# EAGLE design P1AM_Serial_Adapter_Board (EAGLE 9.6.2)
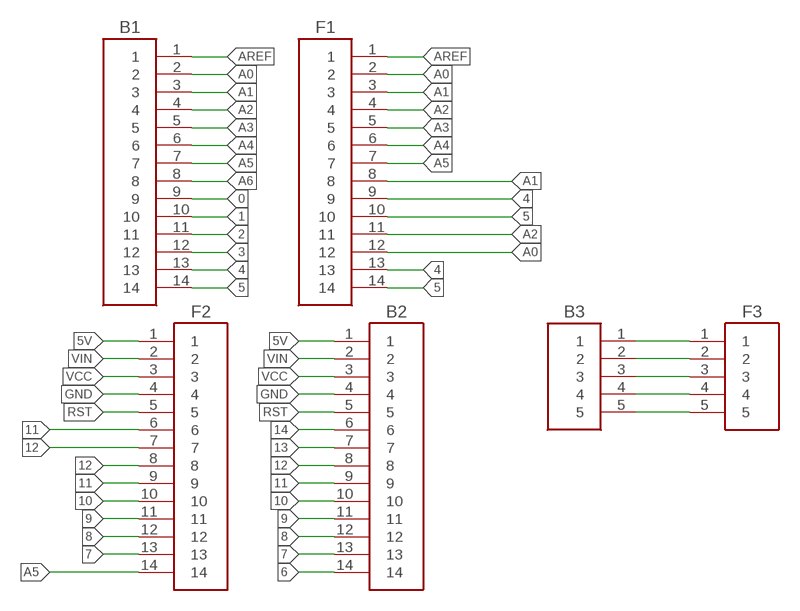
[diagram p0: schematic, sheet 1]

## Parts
B1  14-PN_HDR-2.54  [14-PN_HDR_SMD]
B2  14-PN_HDR-2.54  [14-PN_HDR_SMD]
B3  5-PN_HDR-2.54  [5-PN_HDR_SMD]
F1  14-PN_HDR-2.54  [14-PN_HDR_SMD]
F2  14-PN_HDR-2.54  [14-PN_HDR_SMD]
F3  5-PN_HDR-2.54  [5-PN_HDR_SMD]

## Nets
0: B1.9
1: B1.10
2: B1.11
3: B1.12
4: B1.13 F1.9 F1.13
5: B1.14 F1.10 F1.14
5V: B2.1 F2.1
6: B2.14
7: B2.13 F2.13
8: B2.12 F2.12
9: B2.11 F2.11
10: B2.10 F2.10
11: B2.9 F2.6 F2.9
12: B2.8 F2.7 F2.8
13: B2.7
14: B2.6
A0: B1.2 F1.2 F1.12
A1: B1.3 F1.3 F1.8
A2: B1.4 F1.4 F1.11
A3: B1.5 F1.5
A4: B1.6 F1.6
A5: B1.7 F1.7 F2.14
A6: B1.8
AREF: B1.1 F1.1
GND: B2.4 F2.4
N$1: B3.1 F3.1
N$2: B3.2 F3.2
N$3: B3.3 F3.3
N$4: B3.4 F3.4
N$5: B3.5 F3.5
RST: B2.5 F2.5
VCC: B2.3 F2.3
VIN: B2.2 F2.2

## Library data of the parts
B1 B2 F1 F2 = P1AM:14-PN_HDR-2.54: 2.54mm (0.1") Pitch SIL SMT Pin Header, selective gold + tin, 10 contacts Source: Datasheet
B3 F3 = P1AM:5-PN_HDR-2.54: 2.54mm (0.1") Pitch SIL SMT Pin Header, selective gold + tin, 10 contacts Source: Datasheet

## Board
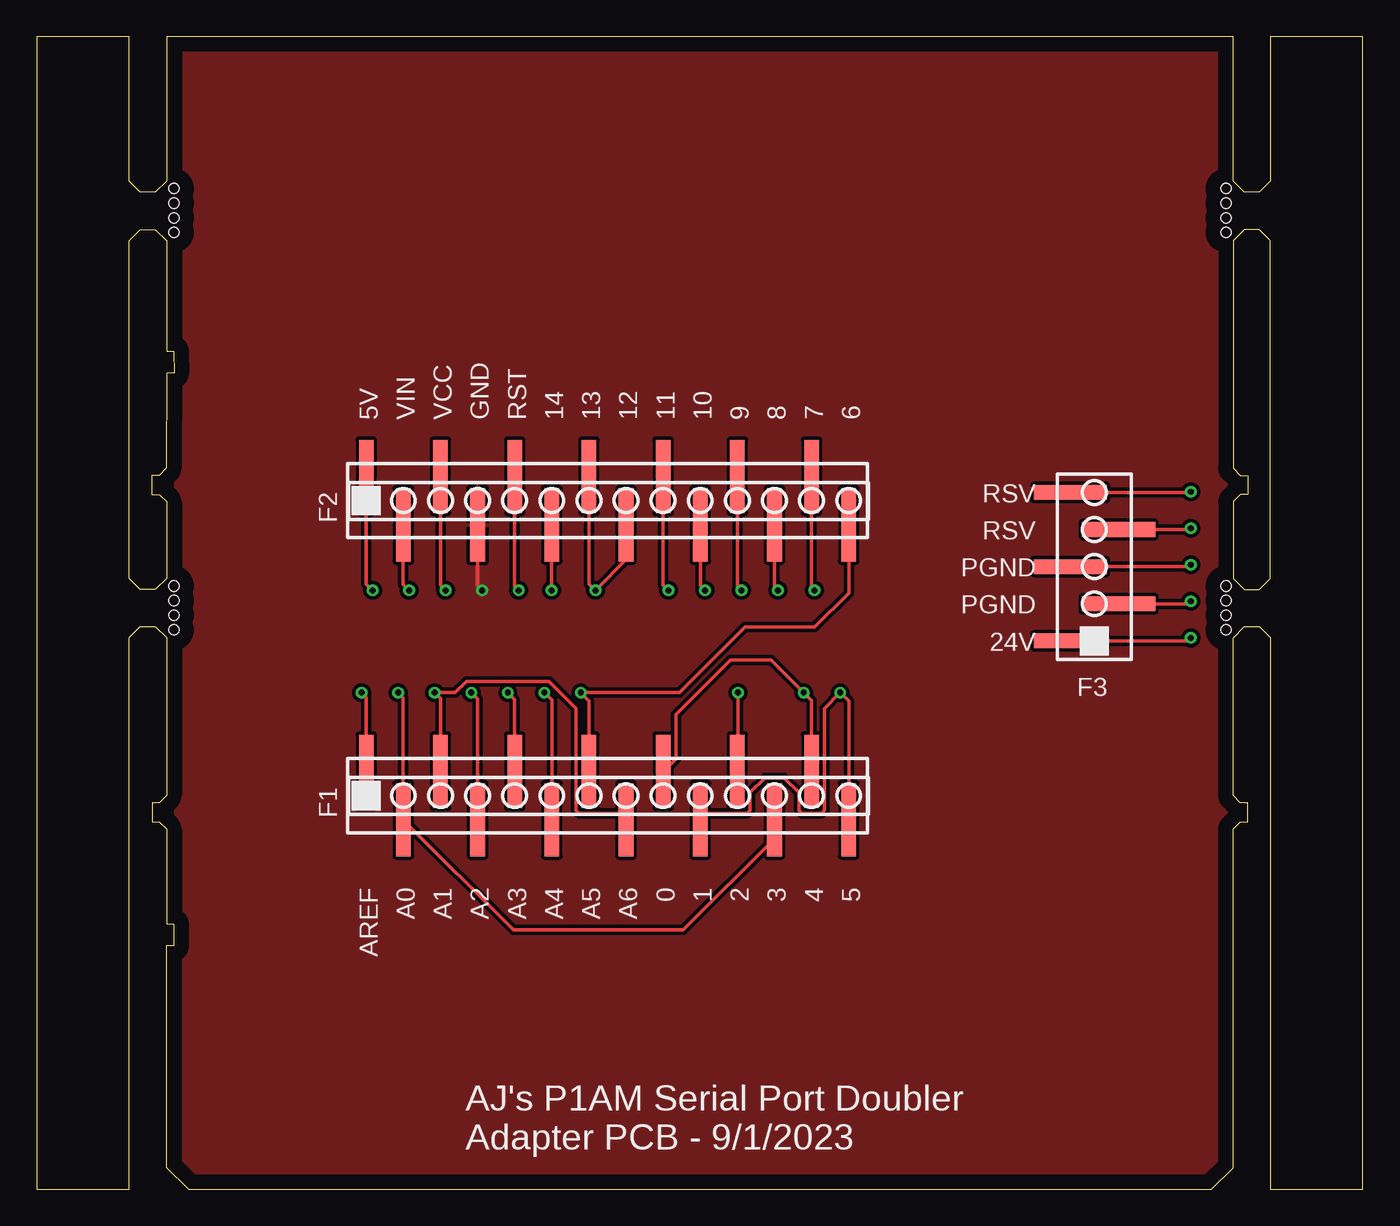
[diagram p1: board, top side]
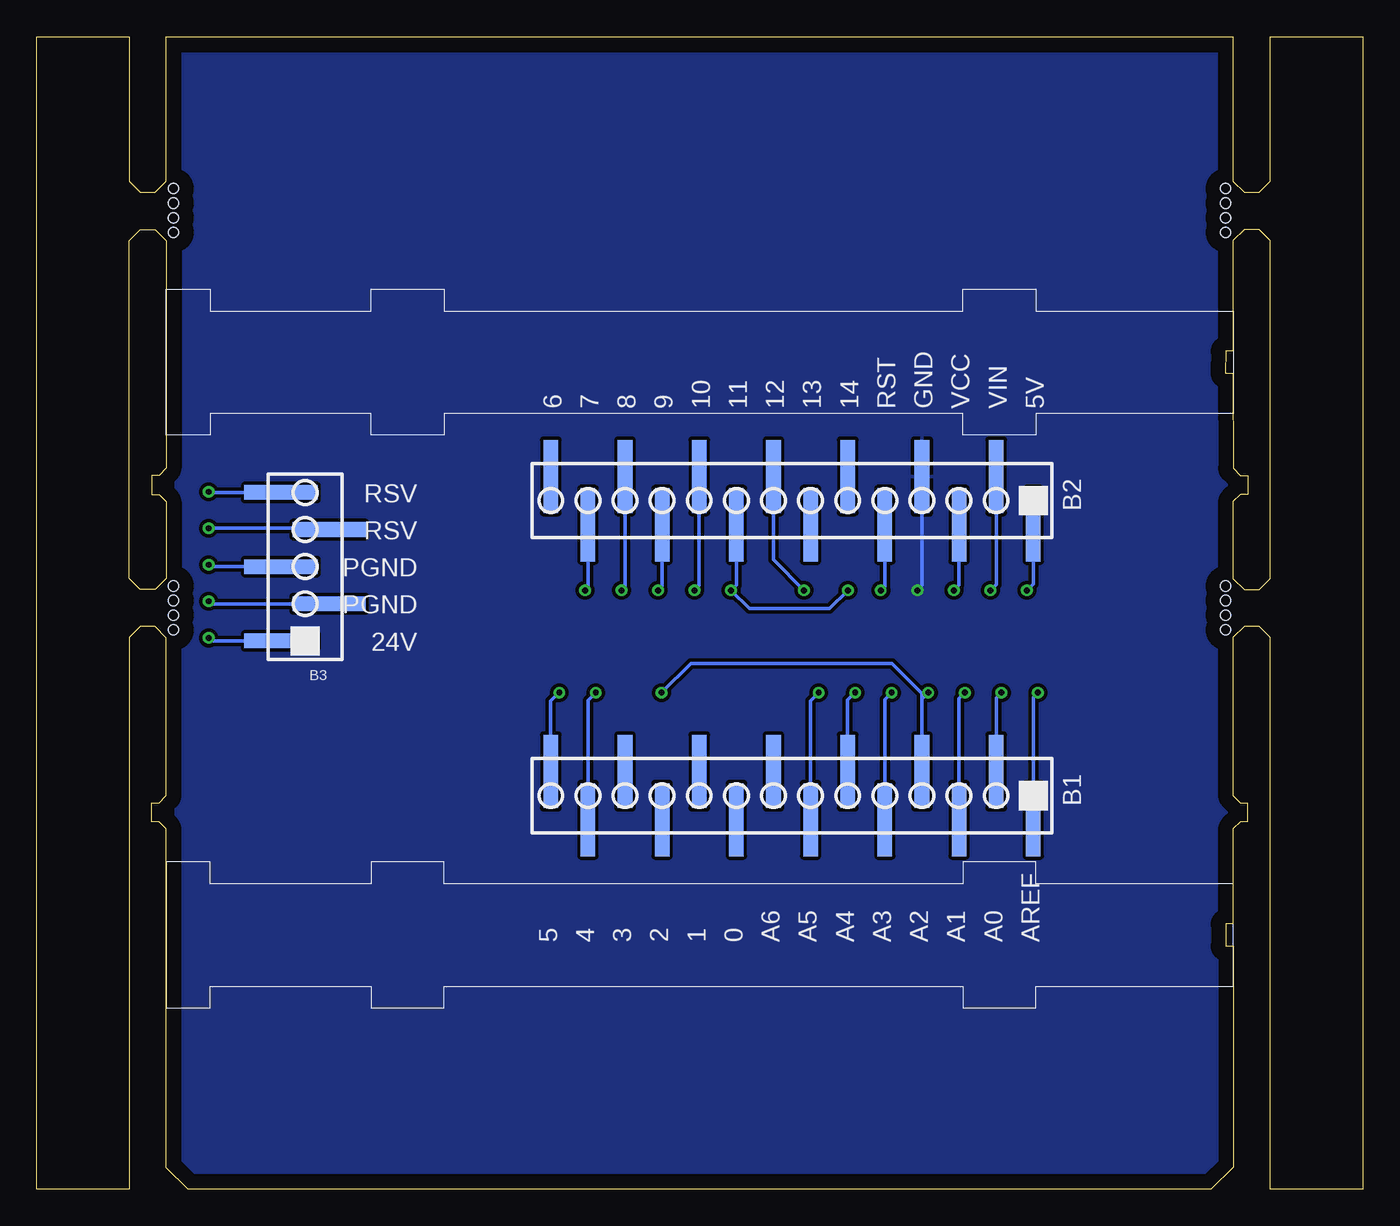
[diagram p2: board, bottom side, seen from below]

Size 90.78 x 78.91 mm. Coordinates in mm from the lower left corner, seen from the top.
Outline: 78 segments
Copper layers (1*16): Top 0.035mm / dielectric 1.5mm / Bottom 0.035mm
Design rules "default *": minimum track width 6mil, minimum drill 0.35mm, track to track 0.24mm, track to pad 0.25mm, pad to pad 0.25mm, via to via 0.25mm, smd to smd 0.2mm, copper to edge 40mil, drill to drill 6mil, minimum pad ring 10mil, minimum via ring 8mil, stop-mask expansion 4mil, vias tented up to drill 0mil, thermal gap 10mil
Holes 0.7 mm at 9.4,68.5 9.4,67.5 9.4,66.5 9.4,65.5 9.4,41.3 9.4,40.3 9.4,39.3 9.4,38.3 81.4,38.3 81.4,39.3 81.4,40.3 81.4,41.3 81.4,65.5 81.4,66.5 81.4,67.5 81.4,68.5

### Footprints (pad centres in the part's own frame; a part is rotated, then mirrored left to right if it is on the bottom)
14-PN_HDR_SMD = smd 1 x 5: 1 0,1.655; 2 2.54,-1.655; 3 5.08,1.655; 4 7.62,-1.655; 5 10.16,1.655; 6 12.7,-1.655; 7 15.24,1.655; 8 17.78,-1.655; 9 20.32,1.655; 10 22.86,-1.655; 11 25.4,1.655; 12 27.94,-1.655; 13 30.48,1.655; 14 33.02,-1.655
5-PN_HDR_SMD = smd 1 x 5: 1 0,1.655; 2 2.54,-1.655; 3 5.08,1.655; 4 7.62,-1.655; 5 10.16,1.655

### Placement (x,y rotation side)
B1  22.57,26.95 180 bottom
B2  22.57,47.14 180 bottom
B3  72.4,37.54 90 bottom
F1  22.57,26.95 0 top
F2  22.57,47.14 0 top
F3  72.4,37.54 90 top

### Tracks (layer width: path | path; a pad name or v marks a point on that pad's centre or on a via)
4  (via drill 0.4)
  Top 0.254: F1.13 53.05,33.45 v52.5,34 50.25,36.25 47.5,36.25 43.75,32.5 43.75,29.47 F1.9
  Bottom 0.254: v52.5,34 53.05,33.45 B1.13
5  (via drill 0.4)
  Top 0.254: F1.14 55.59,33.41 v55,34 53.92,32.92 53.92,25.95 53.7,25.73 52.39,25.73 52.17,25.95 52.17,27.16 51.16,28.17 49.85,28.17 48.84,27.16 48.84,25.95 48.62,25.73 45.86,25.73 F1.10
  Bottom 0.254: v55,34 55.59,33.41 B1.14
5V  (via drill 0.4)
  Top 0.254: v23,41 22.57,41.44 F2.1
  Bottom 0.254: B2.1 22.57,41.44 v23,41
7  (via drill 0.4)
  Top 0.254: F2.13 53.05,41.2 v53.25,41
  Bottom 0.254: v53.25,41 53.05,41.2 B2.13
8  (via drill 0.4)
  Top 0.254: v50.75,41 50.51,41.24 F2.12
  Bottom 0.254: B2.12 50.51,41.24 v50.75,41
9  (via drill 0.4)
  Top 0.254: F2.11 47.97,41.28 v48.25,41
  Bottom 0.254: v48.25,41 47.97,41.28 B2.11
10  (via drill 0.4)
  Top 0.254: v45.75,41 45.42,41.33 F2.10
  Bottom 0.254: B2.10 45.42,41.33 v45.75,41
11  (via drill 0.4)
  Top 0.254: F2.9 42.88,41.37 v43.25,41 | v35.25,41 35.25,45.47 F2.6
  Bottom 0.254: B2.9 42.88,41.37 v43.25,41 42,39.75 36.5,39.75 v35.25,41
12  (via drill 0.4)
  Top 0.254: F2.7 37.8,41.45 v38.25,41 40.34,43.09 F2.8
  Bottom 0.254: v38.25,41 40.34,43.09 B2.8
A0  (via drill 0.4)
  Top 0.254: v24.75,34 25.11,33.65 F1.2 32.65,17.75 44.25,17.75 50.51,24 F1.12
  Bottom 0.254: v24.75,34 25.11,33.65 B1.2
A1  (via drill 0.4)
  Top 0.254: F1.3 27.64,33.6 v27.25,34 28.65,34 29.43,34.78 35.07,34.78 36.93,32.92 36.93,25.95 37.15,25.73 39.91,25.73 F1.8
  Bottom 0.254: B1.3 27.64,33.6 v27.25,34
A2  (via drill 0.4)
  Top 0.254: F1.4 30.18,33.56 v29.75,34 | v48,34 48,28.64 F1.11
  Bottom 0.254: v29.75,34 30.18,33.56 B1.4 30.18,33.94 32.25,36 46,36 v48,34
A3  (via drill 0.4)
  Top 0.254: v32.25,34 32.73,33.52 F1.5
  Bottom 0.254: B1.5 32.73,33.52 v32.25,34
A4  (via drill 0.4)
  Top 0.254: F1.6 35.27,33.48 v34.75,34
  Bottom 0.254: v34.75,34 35.27,33.48 B1.6
A5  (via drill 0.4)
  Top 0.254: F1.7 37.8,33.45 v37.25,34 44,34 48.5,38.5 53.25,38.5 55.59,40.84 F2.14
  Bottom 0.254: B1.7 37.8,33.45 v37.25,34
AREF  (via drill 0.4)
  Top 0.254: v22.25,34 22.57,33.69 F1.1
  Bottom 0.254: B1.1 22.57,33.69 v22.25,34
GND  (via drill 0.4)
  Top 0.254: F2.4 30.18,41.31 v30.5,41
  Bottom 0.254: v30.5,41 30.18,41.31 B2.4
  pour Top: 9.5,78.5 80.75,78.5 81.5,77.75 81.5,69.5 80.5,68.5 80.5,65.5 81.5,64.5 81.5,42.25 80.75,41.5 80.75,38 81.5,37.25 81.5,2 80,0.5 10.75,0.5 9.5,1.75 9.5,37.5 10.25,38.25 10.25,41.5 9.5,42.25 9.5,64.75 10.25,65.5 10.25,68.75 9.5,69.5
  pour Bottom: 81.25,78.25 9.75,78.25 9.25,77.75 9.25,69.5 10.25,68.5 10.25,65.5 9.25,64.5 9.25,42.25 10,41.5 10,38 9.25,37.25 9.25,2 10.75,0.5 80,0.5 81.25,1.75 81.25,37.5 80.5,38.25 80.5,41.5 81.25,42.25 81.25,64.75 80.5,65.5 80.5,68.75 81.25,69.5
N$1  (via drill 0.4)
  Top 0.254: F3.1 78.79,37.54 v79,37.75
  Bottom 0.254: v79,37.75 78.79,37.54 B3.1
N$2  (via drill 0.4)
  Top 0.254: v79,40.25 78.83,40.08 F3.2
  Bottom 0.254: B3.2 78.83,40.08 v79,40.25
N$3  (via drill 0.4)
  Top 0.254: F3.3 78.87,42.62 v79,42.75
  Bottom 0.254: v79,42.75 78.87,42.62 B3.3
N$4  (via drill 0.4)
  Top 0.254: v79,45.25 78.91,45.16 F3.4
  Bottom 0.254: B3.4 70.83,45.25 v79,45.25
N$5  (via drill 0.4)
  Top 0.254: F3.5 78.95,47.7 v79,47.75
  Bottom 0.254: v79,47.75 78.95,47.7 B3.5
RST  (via drill 0.4)
  Top 0.254: v33,41 32.73,41.27 F2.5
  Bottom 0.254: B2.5 32.73,41.27 v33,41
VCC  (via drill 0.4)
  Top 0.254: v28,41 27.64,41.35 F2.3
  Bottom 0.254: B2.3 27.64,41.35 v28,41
VIN  (via drill 0.4)
  Top 0.254: F2.2 25.11,41.4 v25.5,41
  Bottom 0.254: v25.5,41 25.11,41.4 B2.2

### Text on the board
tPlace: 5V / VIN / VCC / GND / RST / 14 / 13 / 12 / 11 / 10 / 9 / 8 / 7 / 6 | RSV / RSV / PGND / PGND / 24V | AREF / A0 / A1 / A2 / A3 / A4 / A5 / A6 / 0 / 1 / 2 / 3 / 4 / 5
tNames: AJ's P1AM Serial Port Doubler / Adapter PCB - 9/1/2023
bNames: 6 / 7 / 8 / 9 / 10 / 11 / 12 / 13 / 14 / RST / GND / VCC / VIN / 5V | RSV / RSV / PGND / PGND / 24V | 5 / 4 / 3 / 2 / 1 / 0 / A6 / A5 / A4 / A3 / A2 / A1 / A0 / AREF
